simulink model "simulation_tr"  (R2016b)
settings: Solver=ode45  StartTime=0.0  StopTime=35*3600  RelTol=1e-3  EnableMultiTasking=on
undefined symbols (not defined in the file or in its folder): C0, C1, drhe, drhi, dte, dti, dto, Icc, Nbre, Qair, Qpanne, R_iso, serial, V, V0, V1
libraries: powerlib_meascontrol x4, instrumentlib x3, simulink x1

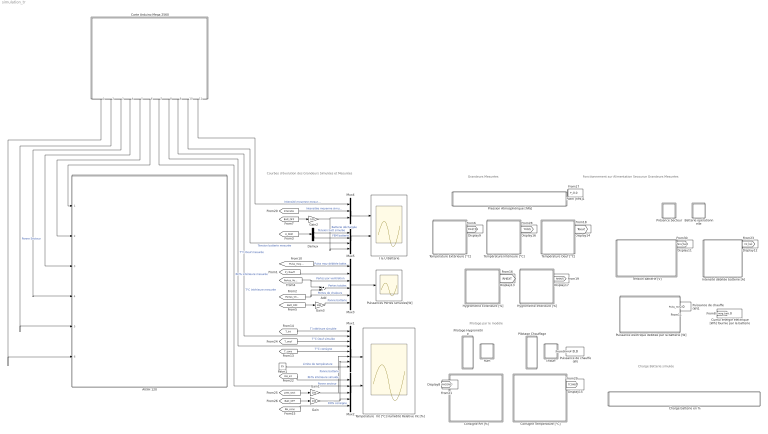
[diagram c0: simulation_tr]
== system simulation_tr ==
  note: Fonctionnement sur Alimentation Secourue Grandeurs Mesurées
  note: Grandeurs Mesurées
  note: Pilotage par le modèle
  note: Courbes d'évolution des Grandeurs Simulées et Mesurées
  note: Charge Batterie simulée
  AVXH 120 : Subsystem
  Add : Sum
  Batterie opérationnelle : Subsystem  DialogController=hmiCreateDDGDialog  IsWebBlock=on
  Carte Arduino Mega 2560 : Subsystem
  Charge batterie en % : Subsystem  DialogController=hmiCreateDDGDialog  IsWebBlock=on
  Consigne RH [%] : Subsystem  DialogController=hmiCreateDDGDialog  IsWebBlock=on
  Consigne Température [°C] : Subsystem  DialogController=hmiCreateDDGDialog  IsWebBlock=on
  Cumul énergie électrique [Wh] fournie par la batterie : Display
  Demux : Demux  Outputs=2
  Display{8..9,11..17} (9 alike) : Display
  Gain{,1..3} (4 alike) : Gain  Gain=100
  Hygrométrie Extérieure [%] : Subsystem  DialogController=hmiCreateDDGDialog  IsWebBlock=on
  Hygrométrie Intérieure [%] : Subsystem  DialogController=hmiCreateDDGDialog  IsWebBlock=on
  I & U Batterie : Scope  NumInputPorts=2
  Intensité débitée batterie [A] : Subsystem  DialogController=hmiCreateDDGDialog  IsWebBlock=on
  Mux1 : Mux  Inputs=8
  Mux2 : Mux  Inputs=5
  Mux3 : Mux  Inputs=6
  Mux4 : Mux  Inputs=3
  Mux5 : Mux
  Patm [hPa]1 : Display
  Patm1 : Constant  Value=25
  Pilotage Chauffage : Subsystem  DialogController=hmiCreateDDGDialog  IsWebBlock=on
  Pilotage Hygrométrie : Subsystem  DialogController=hmiCreateDDGDialog  IsWebBlock=on
  Pression Atmosphérique [hPa] : Subsystem  DialogController=hmiCreateDDGDialog  IsWebBlock=on
  Présence Secteur : Subsystem  DialogController=hmiCreateDDGDialog  IsWebBlock=on
  Puissance de chauffe (W) : Display
  Puissance de chauffe (W)1 : Display
  Puissance électrique débitée par la batterie [W] : Subsystem  DialogController=hmiCreateDDGDialog  IsWebBlock=on
  Puissances Pertes simulées[W] : Scope
  Température Extérieure [°C] : Subsystem  DialogController=hmiCreateDDGDialog  IsWebBlock=on
  Température Intérieure [°C] : Subsystem  DialogController=hmiCreateDDGDialog  IsWebBlock=on
  Température  Int [°C] Humidité Relative Int [%] : Scope  NumInputPorts=2
  Température Oeuf [°C] : Subsystem  DialogController=hmiCreateDDGDialog  IsWebBlock=on
  Tension batterie [V] : Subsystem  DialogController=hmiCreateDDGDialog  IsWebBlock=on
  chauff : Subsystem  DialogController=hmiCreateDDGDialog  IsWebBlock=on
  hum : Subsystem  DialogController=hmiCreateDDGDialog  IsWebBlock=on
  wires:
  [T_int] -> Mux1/1  "T intérieure simulée"
  [Intensite] -> Mux4/2  "Intensitée moyenne simulée"
  [RH_int] -> Mux2/1  "RH% intérieure simulée"
  Gain1/1 -> Mux1/6, Mux2/3  "Panne secteur"
  [pres_sect] -> Gain1/1
  [Batt_OFF] -> Gain/1
  Gain/1 -> Mux1/7, Mux2/4  "Panne batterie"
  Demux/1 -> Mux5/1  "Tension batt simulée"
  [T_cons] -> Mux1/5  "T°C consigne"
  Carte Arduino Mega 2560/1(Patm) -> AVXH 120/6(In6)
  Mux1/1 -> Température  Int [°C] Humidité Relative Int [%]/1
  Mux2/1 -> Température  Int [°C] Humidité Relative Int [%]/2
  [P_chauff] -> Mux3/2
  [Pertes_Vent] -> Mux3/3, Add/1  "Pertes par ventilation"
  Mux3/1 -> Puissances Pertes simulées[W]/1
  [Pertes_Chaleur] -> Mux3/5, Add/2  "Pertes de chaleurs"
  Add/1 -> Mux3/4  "Pertes totales"
  [T_oeuf] -> Mux1/3  "T°C Oeuf simulée"
  Carte Arduino Mega 2560/9(T°C INT) -> Mux1/2  "T°C intérieure mesurée"
  Carte Arduino Mega 2560/7(RH% INT) -> Mux2/2  "RH% intérieure mesurée"
  Carte Arduino Mega 2560/4(RH% EXT) -> AVXH 120/3(In4)
  Carte Arduino Mega 2560/3(T°C EXT) -> AVXH 120/4(In5)
  Carte Arduino Mega 2560/2(Pres Sect) -> AVXH 120/5(Présence secteur)  "Panne Secteur"
  [RH_cons] -> Mux2/5  "RH% consigne"
  Carte Arduino Mega 2560/8(T°C OEUF) -> Mux1/4  "T°C Oeuf mesurée"
  Carte Arduino Mega 2560/5(RH Cons) -> AVXH 120/2(In3)
  Carte Arduino Mega 2560/6(T°C Cons) -> AVXH 120/1(In2)
  [RHCONS] -> Display8/1
  [TCONS] -> Display15/1
  [TCINT] -> Display16/1
  [P_atm] -> Patm [hPa]1/1
  [TCEXT] -> Display9/1
  [Toeuf] -> Display14/1
  [RHINT] -> Display17/1
  [RHEXT] -> Display13/1
  [Int_bat] -> Display12/1
  [Tens_bat] -> Display11/1
  Mux4/1 -> I & U Batterie/1
  Mux5/1 -> I & U Batterie/2
  Carte Arduino Mega 2560/10(U) -> Mux5/3  "Tension batterie mesurée"
  [U_FEM] -> Demux/1
  Demux/2 -> Mux5/2  "FEM batterie"
  [Batt_OFF] -> Gain2/1
  Gain2/1 -> Mux5/4, Mux4/3  "Batterie déchargée"
  [Batt_OFF] -> Gain3/1
  Gain3/1 -> Mux3/6  "Panne batterie"
  [Energ_batt] -> Cumul énergie électrique [Wh] fournie par la batterie/1
  Carte Arduino Mega 2560/11(Imoy) -> Mux4/1  "Intensité moyenne mesurée"
  [Puiss_moy_debitee] -> Mux3/1  "Puiss moy débitée batterie mesurée"
  Patm1/1 -> Mux1/8  "Limite de température"
  [PCHAUFF] -> Puissance de chauffe (W)/1
  [Puiss_moy_debitee] -> Puissance de chauffe (W)1/1

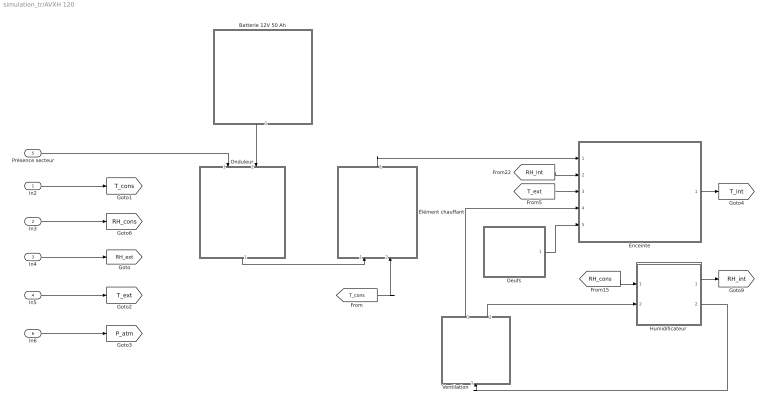
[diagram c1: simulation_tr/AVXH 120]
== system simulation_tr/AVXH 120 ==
  In2 : Inport
  In3 : Inport  Port=2
  In4 : Inport  Port=3
  In5 : Inport  Port=4
  Présence secteur : Inport  Port=5
  In6 : Inport  Port=6
  Batterie 12V 50 Ah : Subsystem
  Enceinte : Subsystem
  Humidificateur : Subsystem
  Oeufs : Subsystem
  Onduleur : Subsystem
  Ventilation : Subsystem
  Élément chauffant : Subsystem
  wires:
  [RH_int] -> Enceinte/2(In2)
  Enceinte/1(T°C in) -> [T_int]
  Présence secteur/1 -> Onduleur/1(In1)
  In6/1 -> [P_atm]
  In5/1 -> [T_ext]
  [T_ext] -> Enceinte/3(T°C ext)
  In4/1 -> [RH_ext]
  In3/1 -> [RH_cons]
  Oeufs/1(Out1) -> Enceinte/5(M.Cp_Oeuf)
  Élément chauffant/1(Out2) -> Enceinte/1(P_chauff)
  Ventilation/1(Out1) -> Enceinte/4(Pertes ventilation)
  [RH_cons] -> Humidificateur/1(In1)
  Ventilation/2(Out2) -> Humidificateur/2(In2)
  Humidificateur/2(Out2) -> Ventilation/1(In1)
  In2/1 -> [T_cons]
  Batterie 12V 50 Ah/1(Out3) -> Onduleur/2(In2)
  Onduleur/1(Out1) -> Élément chauffant/1(In1)
  [T_cons] -> Élément chauffant/2(In2)
  Humidificateur/1(Out1) -> [RH_int]

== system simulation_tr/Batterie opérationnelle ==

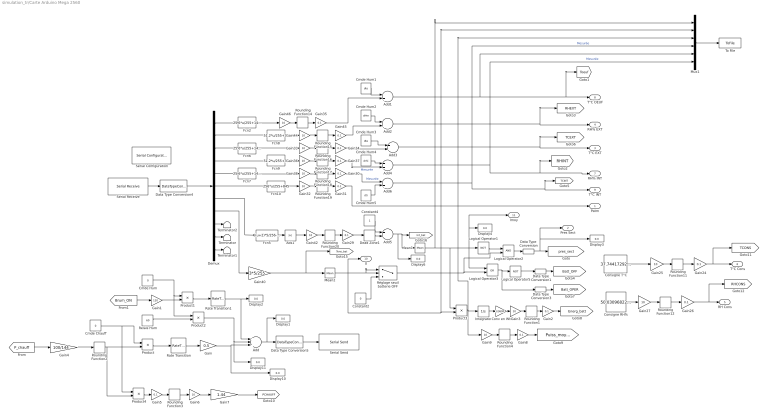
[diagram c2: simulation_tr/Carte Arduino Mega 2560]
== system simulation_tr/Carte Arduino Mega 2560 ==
  Abs1 : Abs
  Add : Sum  Inputs=+++
  Add{1..6} (6 alike) : Sum
  Cmde Chauff : Constant  Value=0  SampleTime=1
  Cmde Hum : Constant  Value=0  SampleTime=1
  Cmde Hum1 : Constant  Value=dto  SampleTime=1
  Cmde Hum2 : Constant  Value=drhe  SampleTime=1
  Cmde Hum3 : Constant  Value=dte  SampleTime=1
  Cmde Hum4 : Constant  Value=drhi  SampleTime=1
  Cmde Hum5 : Constant  Value=dti  SampleTime=1
  Consigne RH% : Constant  Value=50.030968221029
  Consigne T°C : Constant  Value=37.74417292277
  Constant2 : Constant  Value=0
  Constant4 : Constant
  Conv en Wh : Gain  Gain=1/3600
  Data Type Conversion{,1,3..4} (4 alike) : DataTypeConversion  OutDataTypeStr=double
  Data Type Conversion5 : DataTypeConversion  OutDataTypeStr=uint8
  Dead Zone1 : DeadZone  LowerValue=0  UpperValue=1
  Demux : Demux  Outputs=11
  Display{1..4,6,10..11} (7 alike) : Display
  Fcn10 : Fcn  Expr=256*u/255+845
  Fcn2 : Fcn  Expr=25.6*u/255+14.4
  Fcn5 : Fcn  Expr=((u+2)*5/256-2.5)/0.0833
  Fcn6 : Fcn  Expr=25.6*u/255+14.4
  Fcn7 : Fcn  Expr=25.6*u/255+14.4
  Fcn8 : Fcn  Expr=51.2*u/255+35
  Fcn9 : Fcn  Expr=51.2*u/255+35
  Gain : Gain  Gain=0.5
  Gain1 : Gain  Gain=120
  Gain{2,5,8,24,26,29..31,34..35,37,45} (12 alike) : Gain  Gain=0.1
  Gain{3,6,9,25,27,32..33,36,38,42,44,46} (12 alike) : Gain  Gain=10
  Gain4 : Gain  Gain=100/144
  Gain40 : Gain  Gain=3*5/255
  Gain7 : Gain  Gain=1.44
  Integrator : Integrator
  Logical Operator1 : Logic  Operator=NOT  AllPortsSameDT=off  OutDataTypeStr=boolean
  Logical Operator2 : Logic  AllPortsSameDT=off  OutDataTypeStr=boolean
  Logical Operator3 : Logic  Operator=OR  AllPortsSameDT=off  OutDataTypeStr=boolean
  Logical Operator5 : Logic  Operator=NOT  AllPortsSameDT=off  OutDataTypeStr=boolean
  Mean1 : powerlib_meascontrol/Measurements/Mean  Freq=0.1  Vinit=0  Ts=1
  Mean2 : powerlib_meascontrol/Measurements/Mean  Freq=0.1  Vinit=0  Ts=1
  Mux1 : Mux  Inputs=6
  Product{,1..4} (5 alike) : Product
  Rate Transition : RateTransition  OutPortSampleTime=1
  Rate Transition1 : RateTransition  OutPortSampleTime=1
  Relais Hum : Constant  Value=60  SampleTime=1
  Rounding Function{1..4,11..12,14..20} (13 alike) : Rounding  Operator=round
  Réglage seuil batterie OFF : Switch  Criteria=u2 > Threshold  Threshold=11.5
  Serial Configuration : instrumentlib/Serial Configuration  Priority=-200000  ComPortMenu=<Please select a port...>  ComPort=COM8  ObjConstructor=serial('COM8');  BaudRate=9600  DataBits=8  Parity=none  StopBits=1  FlowControl=none  Timeout=10  ByteOrder=LittleEndian
  Serial Receive : instrumentlib/Serial Receive  ComPortMenu=<Please select a port...>  ComPort=COM8  ObjConstructor=serial('COM8');  Terminator=<none>  DataSize="[1  11]"  DataType=uint8  EnableBlockingMode=on  ActionDataUnavailable=Output last received value  CustomValue=0  SampleTime=1
  Serial Send : instrumentlib/Serial Send  ComPortMenu=<Please select a port...>  ComPort=COM8  ObjConstructor=serial('COM8');  Terminator=<none>  EnableBlockingMode=on
  Terminator : Terminator
  Terminator1 : Terminator
  Terminator2 : Terminator
  To File : ToFile  Filename=mesures.mat  SaveFormat=Timeseries
  Patm : Outport
  Pres Sect : Outport  Port=2
  T°C EXT : Outport  Port=3
  RH% EXT : Outport  Port=4
  RH Cons : Outport  Port=5
  T°C Cons : Outport  Port=6
  RH% INT : Outport  Port=7
  T°C OEUF : Outport  Port=8
  T°C INT : Outport  Port=9
  U : Outport  Port=10
  Imoy : Outport  Port=11
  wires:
  Rounding Function11/1 -> Gain24/1
  Gain25/1 -> Rounding Function11/1
  Consigne T°C/1 -> Gain25/1
  Gain24/1 -> [TCONS], T°C Cons/1
  Rounding Function12/1 -> Gain26/1
  Gain27/1 -> Rounding Function12/1
  Gain26/1 -> [RHCONS], RH Cons/1
  Consigne RH%/1 -> Gain27/1
  Mux1/1 -> To File/1
  Add1/1 -> Mux1/5, [Toeuf], T°C OEUF/1
  Add2/1 -> [RHEXT], RH% EXT/1
  Gain31/1 -> Patm/1
  Demux/7 -> Fcn5/1
  Add4/1 -> Mux1/6, RH% INT/1, [RHINT]  "Mesurée"
  Add3/1 -> T°C EXT/1, [TCEXT]
  Gain40/1 -> Mean2/1, [Tens_bat]
  Demux/2 -> Fcn8/1
  Demux/3 -> Fcn6/1
  Demux/4 -> Fcn9/1
  Demux/5 -> Fcn7/1
  Demux/1 -> Fcn2/1
  Fcn2/1 -> Gain46/1
  Fcn6/1 -> Gain33/1
  Fcn7/1 -> Gain38/1
  Fcn8/1 -> Gain44/1
  Fcn9/1 -> Gain36/1
  Fcn10/1 -> Gain32/1
  Rounding Function14/1 -> Gain35/1
  Gain46/1 -> Rounding Function14/1
  Rounding Function15/1 -> Gain45/1
  Gain44/1 -> Rounding Function15/1
  Rounding Function16/1 -> Gain34/1
  Gain33/1 -> Rounding Function16/1
  Rounding Function17/1 -> Gain37/1
  Gain36/1 -> Rounding Function17/1
  Rounding Function18/1 -> Gain30/1
  Gain38/1 -> Rounding Function18/1
  Rounding Function19/1 -> Gain31/1
  Gain32/1 -> Rounding Function19/1
  Serial Receive/1 -> Data Type Conversion4/1
  Data Type Conversion4/1 -> Demux/1
  Rounding Function20/1 -> Gain29/1
  Gain42/1 -> Rounding Function20/1
  Demux/6 -> Fcn10/1
  Add6/1 -> Mux1/4, T°C INT/1, [TCINT]  "Mesurée"
  Fcn5/1 -> Abs1/1
  Gain/1 -> Display10/1, Add/3
  Demux/10 -> Terminator/1
  Demux/11 -> Terminator1/1
  Demux/9 -> Terminator2/1
  Data Type Conversion5/1 -> Serial Send/1
  Rate Transition/1 -> Gain/1
  Constant2/1 -> Réglage seuil batterie OFF/3
  Demux/8 -> Gain40/1
  Réglage seuil batterie OFF/1 -> Logical Operator3/2, Logical Operator2/2
  Data Type Conversion/1 -> Pres Sect/1, Display3/1, [pres_sect]
  Add5/1 -> Display6/1, Mean1/1, [Int_bat]
  Cmde Chauff/1 -> Product4/1, Product/1
  Product/1 -> Rate Transition/1
  Logical Operator2/1 -> Data Type Conversion/1
  Logical Operator3/1 -> Data Type Conversion3/1, Logical Operator5/1
  Logical Operator5/1 -> Data Type Conversion1/1
  Logical Operator1/1 -> Logical Operator2/1
  Data Type Conversion1/1 -> [Batt_OFF]
  Data Type Conversion3/1 -> [Batt_OPER]
  [P_chauff] -> Gain4/1
  Add/1 -> Display1/1, Data Type Conversion5/1
  Cmde Hum/1 -> Product2/1, Product1/1
  [Brum_ON] -> Gain1/1
  Gain1/1 -> Product1/2
  Product1/1 -> Rate Transition1/1
  Rate Transition1/1 -> Display2/1, Add/1
  Relais Hum/1 -> Product2/2
  Product2/1 -> Display11/1, Add/2
  Product3/1 -> Mux1/3, Gain9/1, Integrator/1
  Integrator/1 -> Conv en Wh/1
  Conv en Wh/1 -> Gain3/1
  Rounding Function1/1 -> Gain2/1
  Gain3/1 -> Rounding Function1/1
  Gain2/1 -> [Energ_batt]
  Abs1/1 -> Gain42/1
  Mean1/1 -> Imoy/1, Display4/1, Logical Operator3/1, Logical Operator1/1, Product3/1, Mux1/1
  Mean2/1 -> Réglage seuil batterie OFF/2, Réglage seuil batterie OFF/1, Mux1/2, Product3/2, U/1
  Gain4/1 -> Rounding Function2/1
  Rounding Function2/1 -> Product4/2, Product/2
  Gain5/1 -> Rounding Function3/1
  Rounding Function3/1 -> Gain6/1
  Gain6/1 -> Gain7/1
  Cmde Hum1/1 -> Add1/1
  Gain35/1 -> Add1/2
  Cmde Hum2/1 -> Add2/1
  Gain45/1 -> Add2/2
  Cmde Hum3/1 -> Add3/1
  Gain34/1 -> Add3/2
  Cmde Hum4/1 -> Add4/1
  Gain37/1 -> Add4/2  "Mesurée"
  Cmde Hum5/1 -> Add6/2
  Gain30/1 -> Add6/1  "Mesurée"
  Gain7/1 -> [PCHAUFF]
  Product4/1 -> Gain5/1
  Dead Zone1/1 -> Add5/2
  Constant4/1 -> Add5/1
  Rounding Function4/1 -> Gain8/1
  Gain9/1 -> Rounding Function4/1
  Gain8/1 -> [Puiss_moy_debitee]
  Gain29/1 -> Dead Zone1/1

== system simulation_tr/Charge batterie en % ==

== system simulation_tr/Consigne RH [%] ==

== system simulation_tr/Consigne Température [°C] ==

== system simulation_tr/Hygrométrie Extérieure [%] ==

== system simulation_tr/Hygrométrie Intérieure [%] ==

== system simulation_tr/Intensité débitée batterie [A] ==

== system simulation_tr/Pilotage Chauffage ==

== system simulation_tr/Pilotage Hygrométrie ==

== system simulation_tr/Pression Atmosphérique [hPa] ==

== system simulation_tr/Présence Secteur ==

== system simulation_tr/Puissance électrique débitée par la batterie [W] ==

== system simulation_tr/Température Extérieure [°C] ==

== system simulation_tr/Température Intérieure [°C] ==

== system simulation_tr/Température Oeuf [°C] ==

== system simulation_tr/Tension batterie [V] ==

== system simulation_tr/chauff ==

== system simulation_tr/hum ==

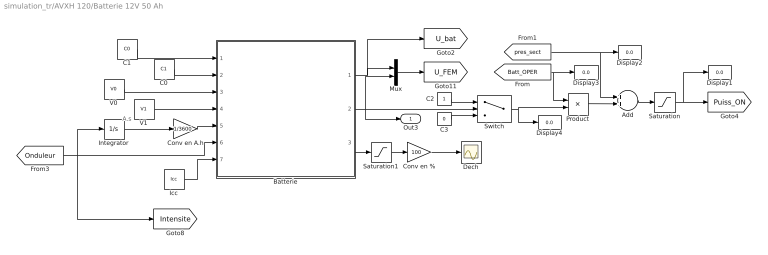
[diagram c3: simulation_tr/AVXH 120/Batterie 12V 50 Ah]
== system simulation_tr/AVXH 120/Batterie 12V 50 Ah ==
  note: A.s
  Add : Sum
  Batterie : MATLAB Function  TreatAsAtomicUnit=on
  C0 : Constant  Value=C1
  C1 : Constant  Value=C0
  C2 : Constant
  C3 : Constant  Value=0
  Conv en % : Gain  Gain=100
  Conv en A.h : Gain  Gain=1/3600
  Dech : Scope
  Display{1..4} (4 alike) : Display
  Icc : Constant  Value=Icc
  Integrator : Integrator
  Mux : Mux  Inputs=2
  Product : Product
  Saturation : Saturate  UpperLimit=1  LowerLimit=0
  Saturation1 : Saturate  UpperLimit=1000  LowerLimit=0
  Switch : Switch  Criteria=u2 > Threshold  Threshold=11
  V0 : Constant  Value=V0
  V1 : Constant  Value=V1
  Out3 : Outport
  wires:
  Batterie/3(x) -> Saturation1/1
  Conv en %/1 -> Dech/1
  Batterie/1(U) -> [U_bat], Mux/1
  C0/1 -> Batterie/2(C1)
  C1/1 -> Batterie/1(C0)
  V0/1 -> Batterie/3(V0)
  V1/1 -> Batterie/4(V1)
  Icc/1 -> Batterie/7(Icc)
  Integrator/1 -> Conv en A.h/1
  Conv en A.h/1 -> Batterie/5(C)
  Mux/1 -> [U_FEM]
  C2/1 -> Switch/1
  C3/1 -> Switch/3
  Saturation1/1 -> Conv en %/1
  Switch/1 -> Display4/1, Product/2
  Product/1 -> Add/2
  [Batt_OPER] -> Display3/1, Product/1
  Add/1 -> Saturation/1
  [pres_sect] -> Display2/1, Add/1
  Batterie/2(E) -> Mux/2, Out3/1, Switch/2
  Saturation/1 -> Display1/1, [Puiss_ON]
  [Onduleur] -> [Intensite], Integrator/1, Batterie/6(I)

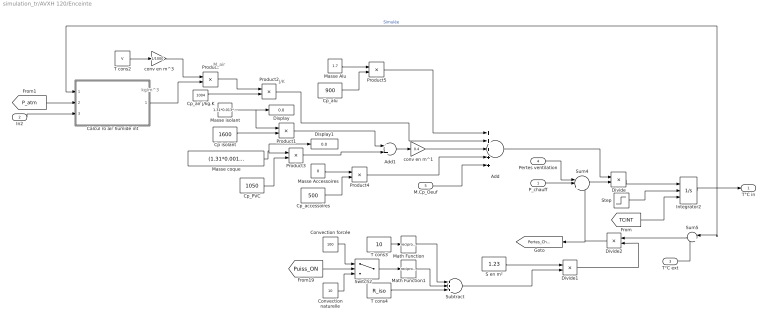
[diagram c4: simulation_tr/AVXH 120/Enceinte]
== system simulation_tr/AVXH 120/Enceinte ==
  note: J/K
  note: kg/m^3
  note: M_air
  P_chauff : Inport
  In2 : Inport  Port=2
  T°C ext : Inport  Port=3
  Pertes ventilation : Inport  Port=4
  M.Cp_Oeuf : Inport  Port=5
  Add : Sum  Inputs=+++++
  Add1 : Sum
  Calcul ro air humide int : MATLAB Function  TreatAsAtomicUnit=on
  Convection forcée : Constant  Value=100
  Convection naturelle : Constant  Value=10
  Cp isolant : Constant  Value=1600
  Cp_PVC : Constant  Value=1050
  Cp_accessoires : Constant  Value=500
  Cp_air j/kg.K : Constant  Value=1004
  Cp_alu : Constant  Value=900
  Display : Display
  Display1 : Display
  Divide : Product  Inputs=/*
  Divide1 : Product  Inputs=*/
  Divide2 : Product  Inputs=**
  Integrator2 : Integrator  ExternalReset=rising  InitialConditionSource=external  InitialCondition=20
  Masse Accessoires : Constant  Value=8
  Masse Alu : Constant  Value=1.7
  Masse coque : Constant  Value=(1.31*0.001+1.23*0.001)*1380
  Masse isolant : Constant  Value=1.31*0.013*40
  Math Function : Math  Operator=reciprocal
  Math Function1 : Math  Operator=reciprocal
  Product{,1..5} (6 alike) : Product
  S en m² : Constant  Value=1.23
  Step : Step  SampleTime=0
  Subtract : Sum  Inputs=+++
  Sum4 : Sum  Inputs=-|+|-
  Sum5 : Sum  Inputs=|+-
  Switch2 : Switch  Criteria=u2 > Threshold
  T cons2 : Constant  Value=V
  T cons3 : Constant  Value=10
  T cons4 : Constant  Value=R_iso
  conv en m^1 : Gain  Gain=0.4
  conv en m^3 : Gain  Gain=1/1000
  T°C in : Outport
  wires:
  P_chauff/1 -> Sum4/2
  Sum4/1 -> Divide/2
  Sum5/1 -> Divide2/1
  Divide2/1 -> Sum4/3, [Pertes_Chaleur]
  Divide/1 -> Integrator2/1
  T°C ext/1 -> Sum5/2
  T cons2/1 -> conv en m^3/1
  Calcul ro air humide int/1(RO) -> Product/2
  Product/1 -> Product2/1
  Masse isolant/1 -> Display/1, Product1/1
  Cp_air j/kg.K/1 -> Product2/2
  Cp isolant/1 -> Product1/2
  Product1/1 -> Add1/1
  Product2/1 -> Add/2
  [P_atm] -> Calcul ro air humide int/2(P)
  Add/1 -> Divide/1
  S en m²/1 -> Divide1/1
  T cons4/1 -> Subtract/3
  Divide1/1 -> Divide2/2
  In2/1 -> Calcul ro air humide int/3(RH)
  Pertes ventilation/1 -> Sum4/1
  conv en m^3/1 -> Product/1
  T cons3/1 -> Math Function/1
  Switch2/1 -> Math Function1/1
  Math Function1/1 -> Subtract/2
  Math Function/1 -> Subtract/1
  Subtract/1 -> Divide1/2
  Cp_PVC/1 -> Product3/2
  Product3/1 -> Add1/2
  Masse Accessoires/1 -> Product4/1
  Cp_accessoires/1 -> Product4/2
  Product4/1 -> Add/4
  Masse Alu/1 -> Product5/1
  Cp_alu/1 -> Product5/2
  Product5/1 -> Add/1
  M.Cp_Oeuf/1 -> Add/5
  [TCINT] -> Integrator2/3
  Masse coque/1 -> Display1/1, Product3/1
  Integrator2/1 -> Sum5/1, Calcul ro air humide int/1(T), T°C in/1  "Simulée"
  Add1/1 -> conv en m^1/1
  conv en m^1/1 -> Add/3
  Convection forcée/1 -> Switch2/1
  Convection naturelle/1 -> Switch2/3
  [Puiss_ON] -> Switch2/2
  Step/1 -> Integrator2/2

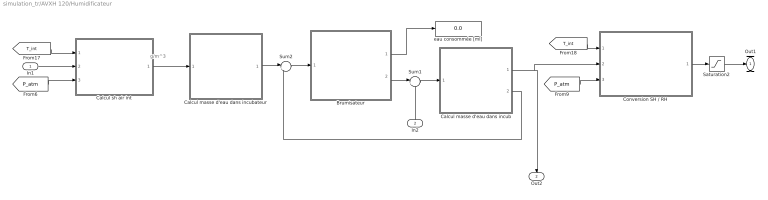
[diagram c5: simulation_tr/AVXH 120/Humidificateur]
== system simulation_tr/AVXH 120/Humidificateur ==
  note: g/m^3
  In1 : Inport
  In2 : Inport  Port=2
  Brumisateur : Subsystem
  Calcul masse d'eau dans incub : Subsystem
  Calcul masse d'eau dans incubateur : Subsystem
  Calcul sh air int : MATLAB Function  TreatAsAtomicUnit=on
  Conversion SH / RH : MATLAB Function  TreatAsAtomicUnit=on
  Saturation2 : Saturate  UpperLimit=100  LowerLimit=0
  Sum1 : Sum  Inputs=|++
  Sum2 : Sum  Inputs=|+-
  eau consommée [ml] : Display
  Out1 : Outport
  Out2 : Outport  Port=2
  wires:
  Sum2/1 -> Brumisateur/1(In1)
  [P_atm] -> Calcul sh air int/3(pl)
  Conversion SH / RH/1(rh) -> Saturation2/1
  Brumisateur/2(Out2) -> Sum1/1
  In1/1 -> Calcul sh air int/2(rh)
  Calcul sh air int/1(sh) -> Calcul masse d'eau dans incubateur/1(In1)
  Calcul masse d'eau dans incub/1(Out1) -> Out2/1, Conversion SH / RH/2(sh)
  Sum1/1 -> Calcul masse d'eau dans incub/1(In1)
  [T_int] -> Calcul sh air int/1(T)
  Calcul masse d'eau dans incubateur/1(Out1) -> Sum2/1
  In2/1 -> Sum1/2
  [T_int] -> Conversion SH / RH/1(T)
  [P_atm] -> Conversion SH / RH/3(pl)
  Brumisateur/1(Q eau consommée (ml)) -> eau consommée [ml]/1
  Calcul masse d'eau dans incub/2(Out2) -> Sum2/2
  Saturation2/1 -> Out1/1

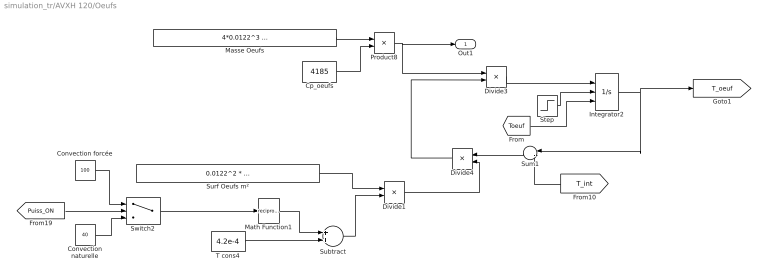
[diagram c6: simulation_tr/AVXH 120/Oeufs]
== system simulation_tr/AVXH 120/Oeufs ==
  Convection forcée : Constant  Value=100
  Convection naturelle : Constant  Value=40
  Cp_oeufs : Constant  Value=4185
  Divide1 : Product  Inputs=*/
  Divide3 : Product  Inputs=/*
  Divide4 : Product  Inputs=**
  Integrator2 : Integrator  ExternalReset=rising  InitialConditionSource=external  InitialCondition=20
  Masse Oeufs : Constant  Value=4*0.0122^3 * (3.14 * (3 - 1.4142) - 1) * 1000 * Nbre / 3
  Math Function1 : Math  Operator=reciprocal
  Product8 : Product
  Step : Step  SampleTime=0
  Subtract : Sum
  Sum1 : Sum  Inputs=|-+
  Surf Oeufs m² : Constant  Value=0.0122^2 * (3.14 * (3 - 1.4142) - 1) * Nbre
  Switch2 : Switch  Criteria=u2 > Threshold  Threshold=0.5
  T cons4 : Constant  Value=4.2e-4
  Out1 : Outport
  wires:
  Cp_oeufs/1 -> Product8/2
  Masse Oeufs/1 -> Product8/1
  Product8/1 -> Out1/1, Divide3/1
  Divide4/1 -> Divide3/2
  [Toeuf] -> Integrator2/3
  Integrator2/1 -> [T_oeuf], Sum1/1
  Sum1/1 -> Divide4/1
  T cons4/1 -> Subtract/2
  Divide1/1 -> Divide4/2
  Math Function1/1 -> Subtract/1
  Subtract/1 -> Divide1/2
  [T_int] -> Sum1/2
  Divide3/1 -> Integrator2/1
  Surf Oeufs m²/1 -> Divide1/1
  Convection forcée/1 -> Switch2/1
  Convection naturelle/1 -> Switch2/3
  [Puiss_ON] -> Switch2/2
  Switch2/1 -> Math Function1/1
  Step/1 -> Integrator2/2

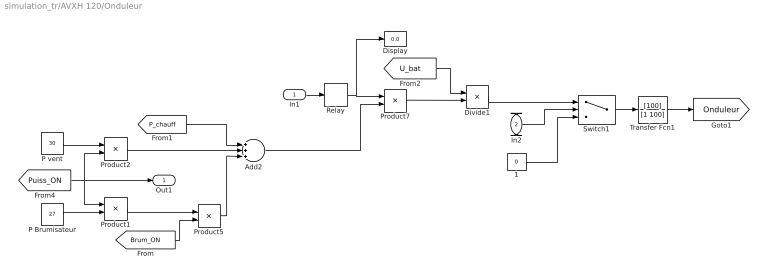
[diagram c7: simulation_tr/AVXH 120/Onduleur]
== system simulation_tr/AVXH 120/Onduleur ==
  In1 : Inport
  In2 : Inport  Port=2
  1 : Constant  Value=0
  Add2 : Sum  Inputs=+++
  Display : Display
  Divide1 : Product  Inputs=/*
  P Brumisateur : Constant  Value=27
  P vent : Constant  Value=30
  Product{1..2,5,7} (4 alike) : Product
  Relay : Relay  OnSwitchValue=1  OffSwitchValue=0  OnOutputValue=0  OffOutputValue=1
  Switch1 : Switch  Threshold=11
  Transfer Fcn1 : TransferFcn  Numerator=[100]  Denominator=[1 100]
  Out1 : Outport
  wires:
  Relay/1 -> Display/1, Product7/1
  Add2/1 -> Product7/2
  Product2/1 -> Add2/2
  [Brum_ON] -> Product5/2
  P Brumisateur/1 -> Product1/2
  Product5/1 -> Add2/3
  In1/1 -> Relay/1
  [P_chauff] -> Add2/1
  Divide1/1 -> Switch1/1
  1/1 -> Switch1/3
  Product7/1 -> Divide1/2
  [U_bat] -> Divide1/1
  Switch1/1 -> Transfer Fcn1/1
  In2/1 -> Switch1/2
  [Puiss_ON] -> Product1/1, Out1/1, Product2/2
  Product1/1 -> Product5/1
  P vent/1 -> Product2/1
  Transfer Fcn1/1 -> [Onduleur]

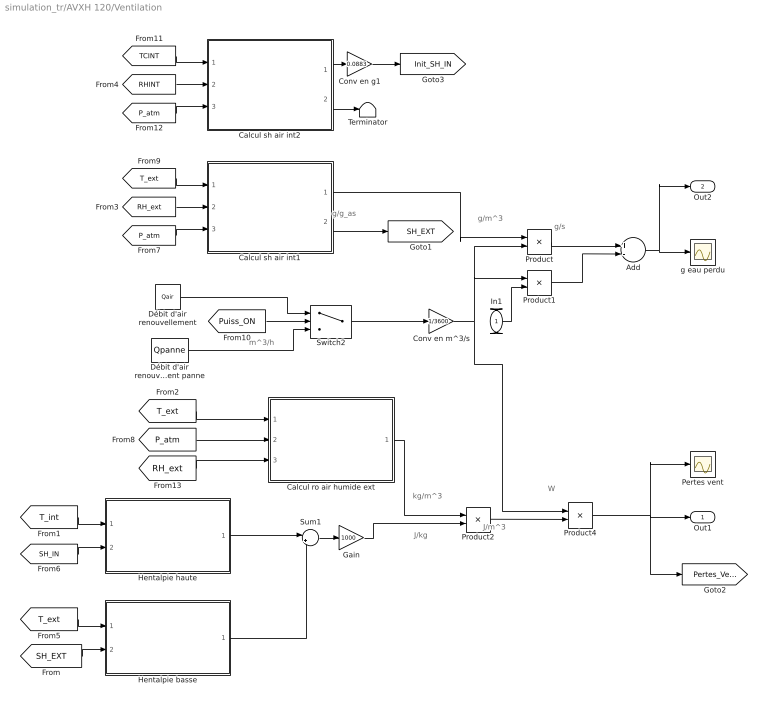
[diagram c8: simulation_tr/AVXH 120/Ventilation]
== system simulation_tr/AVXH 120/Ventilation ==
  note: g/g_as
  note: g/s
  note: W
  note: J/m^3
  note: kg/m^3
  note: J/kg
  note: g/m^3
  note: m^3/h
  In1 : Inport
  Add : Sum  Inputs=+-
  Calcul ro air humide ext : MATLAB Function  TreatAsAtomicUnit=on
  Calcul sh air int1 : MATLAB Function  TreatAsAtomicUnit=on
  Calcul sh air int2 : MATLAB Function  TreatAsAtomicUnit=on
  Conv en g1 : Gain  Gain=0.0883
  Conv en m^3/s : Gain  Gain=1/3600
  Débit d'air renouvellement : Constant  Value=Qair
  Débit d'air renouvellement panne : Constant  Value=Qpanne
  Gain : Gain  Gain=1000
  Hentalpie basse : MATLAB Function  TreatAsAtomicUnit=on
  Hentalpie haute : MATLAB Function  TreatAsAtomicUnit=on
  Pertes vent : Scope
  Product{,1..2,4} (4 alike) : Product
  Sum1 : Sum  Inputs=|+-
  Switch2 : Switch  Criteria=u2 > Threshold
  Terminator : Terminator
  g eau perdu : Scope
  Out1 : Outport
  Out2 : Outport  Port=2
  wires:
  Add/1 -> Out2/1, g eau perdu/1
  Switch2/1 -> Conv en m^3/s/1
  Conv en m^3/s/1 -> Product1/1, Product/2, Product4/1
  Product/1 -> Add/1
  Product1/1 -> Add/2
  Calcul ro air humide ext/1(RO) -> Product2/1
  Product2/1 -> Product4/2
  Débit d'air renouvellement/1 -> Switch2/1
  Débit d'air renouvellement panne/1 -> Switch2/3
  [Puiss_ON] -> Switch2/2
  [T_ext] -> Calcul ro air humide ext/1(T)
  [T_ext] -> Calcul sh air int1/1(T)
  [P_atm] -> Calcul sh air int1/3(pl)
  [P_atm] -> Calcul ro air humide ext/2(P)
  [RH_ext] -> Calcul sh air int1/2(rh)
  [RH_ext] -> Calcul ro air humide ext/3(RH)
  Product4/1 -> [Pertes_Vent], Out1/1, Pertes vent/1
  In1/1 -> Product1/2
  Gain/1 -> Product2/2
  [T_int] -> Hentalpie haute/1(T)
  [T_ext] -> Hentalpie basse/1(T)
  [SH_EXT] -> Hentalpie basse/2(SH)
  [SH_IN] -> Hentalpie haute/2(SH)
  Hentalpie haute/1(H1) -> Sum1/1
  Hentalpie basse/1(H1) -> Sum1/2
  Sum1/1 -> Gain/1
  Calcul sh air int1/2(sh2) -> [SH_EXT]
  [RHINT] -> Calcul sh air int2/2(rh)
  [TCINT] -> Calcul sh air int2/1(T)
  [P_atm] -> Calcul sh air int2/3(pl)
  Calcul sh air int2/1(sh) -> Conv en g1/1
  Conv en g1/1 -> [Init_SH_IN]
  Calcul sh air int1/1(sh) -> Product/1
  Calcul sh air int2/2(sh2) -> Terminator/1

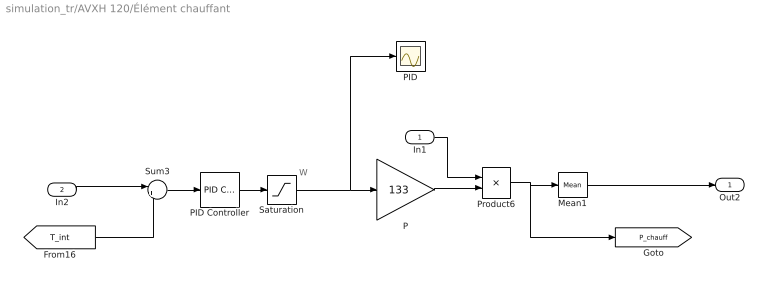
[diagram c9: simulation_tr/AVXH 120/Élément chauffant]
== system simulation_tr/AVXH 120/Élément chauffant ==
  note: W
  In1 : Inport
  In2 : Inport  Port=2
  Mean1 : powerlib_meascontrol/Measurements/Mean  Freq=0.1  Vinit=0  Ts=1
  P : Gain  Gain=133
  PID : Scope
  PID Controller : simulink/Continuous/PID Controller  Controller=PID  TimeDomain=Continuous-time  SampleTime=-1  IntegratorMethod=Forward Euler  FilterMethod=Forward Euler  Form=Parallel  UseFilter=on  ControllerParametersSource=internal  P=0.0897573355031779  I=3.41688472569394e-05  D=-22.2891464593491  N=0.00402695256486726  InitialConditionSource=internal  InitialConditionForIntegrator=0  InitialConditionForFilter=0  ExternalReset=none  LimitOutput=off  UpperSaturationLimit=inf  LowerSaturationLimit=-inf  LinearizeAsGain=on  AntiWindupMode=none  Kb=1  TrackingMode=off  Kt=1  PParamMin=[]  PParamMax=[]  IParamMin=[]  IParamMax=[]  DParamMin=[]  DParamMax=[]  NParamMin=[]  NParamMax=[]  KbParamMin=[]  KbParamMax=[]  KtParamMin=[]  KtParamMax=[]  POutMin=[]  POutMax=[]  IOutMin=[]  IOutMax=[]  DOutMin=[]  DOutMax=[]  NOutMin=[]  NOutMax=[]  KbOutMin=[]  KbOutMax=[]  KtOutMin=[]  KtOutMax=[]  IntegratorOutMin=[]  IntegratorOutMax=[]  FilterOutMin=[]  FilterOutMax=[]  SumOutMin=[]  SumOutMax=[]  SumI1OutMin=[]  SumI1OutMax=[]  SumI2OutMin=[]  SumI2OutMax=[]  SumI3OutMin=[]  SumI3OutMax=[]  SumDOutMin=[]  SumDOutMax=[]  SaturationOutMin=[]  SaturationOutMax=[]  IntegratorContinuousStateAttributes=''  IntegratorStateMustResolveToSignalObject=off  IntegratorRTWStateStorageClass=Auto  FilterContinuousStateAttributes=''  FilterStateMustResolveToSignalObject=off  FilterRTWStateStorageClass=Auto  DifferentiatorICPrevScaledInput=0  DifferentiatorOutMin=[]  DifferentiatorOutMax=[]
  Product6 : Product
  Saturation : Saturate  UpperLimit=1  LowerLimit=0
  Sum3 : Sum  Inputs=|+-
  Out2 : Outport
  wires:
  In2/1 -> Sum3/1
  PID Controller/1 -> Saturation/1
  Sum3/1 -> PID Controller/1
  Product6/1 -> Mean1/1, [P_chauff]
  [T_int] -> Sum3/2
  In1/1 -> Product6/1
  P/1 -> Product6/2
  Saturation/1 -> P/1, PID/1
  Mean1/1 -> Out2/1

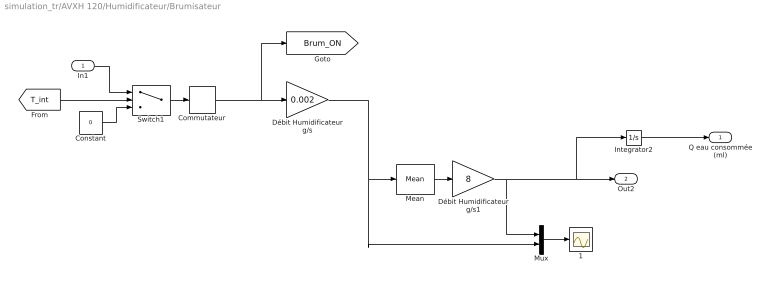
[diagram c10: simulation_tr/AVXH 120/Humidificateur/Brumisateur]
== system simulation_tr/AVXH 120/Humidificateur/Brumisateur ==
  In1 : Inport
  1 : Scope
  Commutateur : Relay  OnSwitchValue=0.11  OffSwitchValue=-0.02
  Constant : Constant  Value=0
  Débit Humidificateur g/s : Gain  Gain=0.002
  Débit Humidificateur g/s1 : Gain  Gain=8
  Integrator2 : Integrator
  Mean : powerlib_meascontrol/Measurements/Mean  Freq=0.061  Vinit=0  Ts=0
  Mux : Mux  Inputs=2
  Switch1 : Switch  Criteria=u2 > Threshold  Threshold=25
  Q eau consommée (ml) : Outport
  Out2 : Outport  Port=2
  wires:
  Integrator2/1 -> Q eau consommée (ml)/1
  Commutateur/1 -> Débit Humidificateur g/s/1, [Brum_ON]
  In1/1 -> Switch1/1
  Débit Humidificateur g/s/1 -> Mux/2, Mean/1
  Mux/1 -> 1/1
  Mean/1 -> Débit Humidificateur g/s1/1
  Débit Humidificateur g/s1/1 -> Mux/1, Integrator2/1, Out2/1
  Switch1/1 -> Commutateur/1
  [T_int] -> Switch1/2
  Constant/1 -> Switch1/3

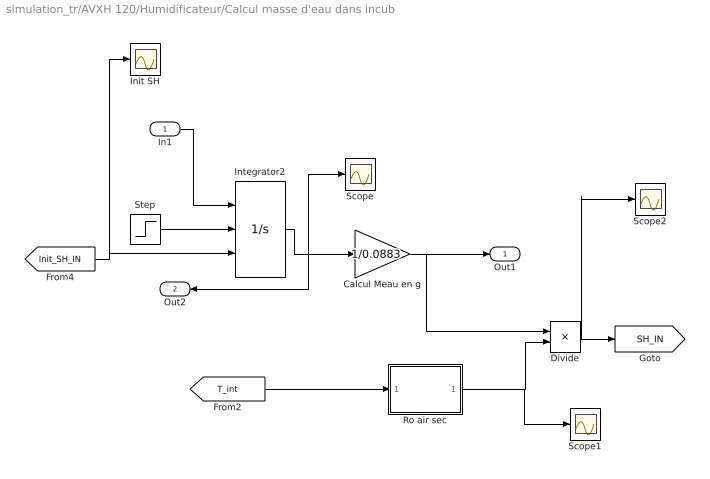
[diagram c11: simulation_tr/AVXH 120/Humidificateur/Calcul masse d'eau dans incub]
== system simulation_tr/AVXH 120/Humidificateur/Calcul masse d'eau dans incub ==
  In1 : Inport
  Calcul Meau en g : Gain  Gain=1/0.0883
  Divide : Product  Inputs=*/
  Init SH : Scope
  Integrator2 : Integrator  ExternalReset=rising  InitialConditionSource=external  InitialCondition=1
  Ro air sec : MATLAB Function  TreatAsAtomicUnit=on
  Scope : Scope
  Scope1 : Scope
  Scope2 : Scope
  Step : Step  SampleTime=0
  Out1 : Outport
  Out2 : Outport  Port=2
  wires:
  Calcul Meau en g/1 -> Divide/1, Out1/1
  In1/1 -> Integrator2/1
  Integrator2/1 -> Scope/1, Calcul Meau en g/1, Out2/1
  Ro air sec/1(ro) -> Scope1/1, Divide/2
  [T_int] -> Ro air sec/1(T)
  Divide/1 -> Scope2/1, [SH_IN]
  [Init_SH_IN] -> Init SH/1, Integrator2/3
  Step/1 -> Integrator2/2

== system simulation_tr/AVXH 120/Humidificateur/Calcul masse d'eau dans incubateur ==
  In1 : Inport
  Calcul Masse eau dans Incub en g : Gain  Gain=0.0883
  Out1 : Outport
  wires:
  In1/1 -> Calcul Masse eau dans Incub en g/1
  Calcul Masse eau dans Incub en g/1 -> Out1/1

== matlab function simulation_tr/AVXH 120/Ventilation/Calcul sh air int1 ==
function [sh,sh2] =CONV_RH_en_SH(T,rh,pl)

% ######################################################################################################
% function [sh]=goff_gratch(T,rh,pl)
%
% fonction de conversion de l'humidité relative ('rh' : en %)
% en humidité spécifique ('sh' : en g/m^3)
% en fonction de :
% la temperature de l'air ('T' : Kelvin, utiliser la fonction C2K si la T est en °C)
% du niveau pression ('pl' : en hPa, si vous avez des matrices 4D, bouclez sur la dimension 
% niveau). 
%
% utilise l'equation de Goff-Gratch pour la determination de
% la tension de vapeur saturante (es) en fonction de la temperature de l'Air
%
% AUTHOR : Nicolas Fauchereau - CRC Dijon - <nicolasf@u-bourgogne.fr>
%
% ######################################################################################################



%Conversion température
T=T+273;


% tension de vapeur saturante
if (T<0), % par rapport a la glace 
eilog = -9.09718 .* ((273.16 ./ T) -1);
eilog2 = -3.5654 .* log10 (273.16 ./ T);
eilog3 = 0.876793 .* (1 - (T ./ 273.16 ));
es=6.1071 .* 10.^(eilog+eilog2+eilog3);

else, % par rapport à l'eau 
eilog=-7.90298 .* ((373.16 ./ T) - 1);
eilog2=5.02808 .* log10((373.16 ./ T));
eilog3=-1.3816e-7 .* ((10.^(11.344.*(1-(T./373.16)))) -1);
eilog4=8.1328e-3 .* ((10.^( -3.49149 .* ((373.16 ./ T) - 1) )) -1);
es=1013.246 .* 10.^(eilog+eilog2+eilog3+eilog4);
end;


% masse
ws = 0.62197 .* es ./ (pl - 0.378.*es);

% masse volumique
ro = 1.293 .* 273 ./ (T);

% humidité spécifique
sh2 = (rh/100.0) .* ws*1000;
sh=sh2*ro; %%% passage en g.m^3

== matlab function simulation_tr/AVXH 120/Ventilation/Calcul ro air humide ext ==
function RO = RO_AIR_HUMIDE(T,P,RH)
P=P*100;
RH=RH/100;
RO = 1/(287.06*(T+273.15))*(P-230.617*RH*exp(17.5043*T/(241.2+T)));

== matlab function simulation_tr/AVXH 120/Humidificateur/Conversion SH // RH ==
function rh  = CONV_SH_en_RH(T,sh,pl)

% ######################################################################################################
% function [sh]=goff_gratch_shtorh(T,sh,pl)
%
% fonction de conversion de l'humidité spécifique ('sh' : en g/m^3)
% en humidité relative ('rh' : %)
% en fonction de :
% la temperature de l'air ('T' : Kelvin, utiliser la fonction C2K si la T est en °C)
% du niveau pression ('pl' : en hPa, si vous avez des matrices 4D, bouclez sur la dimension
% niveau).
%
% utilise l'equation de Goff-Gratch pour la determination de
% la tension de vapeur saturante (es) en fonction de la temperature de l'Air
%
% AUTHOR : Nicolas Fauchereau - CRC Dijon - <nicolasf@u-bourgogne.fr>
%
% ######################################################################################################

%Conversion température
T=T+273;

% tension de vapeur saturante
%if (K2C(T)<0), % par rapport a la glace
if (T<0),
eilog = -9.09718 .* ((273.16 ./ T) -1);
eilog2 = -3.5654 .* log10 (273.16 ./ T);
eilog3 = 0.876793 .* (1 - (T ./ 273.16 ));
es=6.1071 .* 10.^(eilog+eilog2+eilog3);

else, % par rapport à l'eau
eilog=-7.90298 .* ((373.16 ./ T) - 1);
eilog2=5.02808 .* log10((373.16 ./ T));
eilog3=-1.3816e-7 .* ((10.^(11.344.*(1-(T./373.16)))) -1);
eilog4=8.1328e-3 .* ((10.^( -3.49149 .* ((373.16 ./ T) - 1) )) -1);
es=1013.246 .* 10.^(eilog+eilog2+eilog3+eilog4);
end;


% masse
ws = 0.62197 .* es ./ (pl - 0.378.*es);

% masse volumique
ro = 1.293 .* 273 ./ (T);

% humidité relative
rh=(sh./ws) .* 100/(1000*ro);

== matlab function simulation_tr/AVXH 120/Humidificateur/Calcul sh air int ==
function sh =CONV_RH_en_SH(T,rh,pl)

% ######################################################################################################
% function [sh]=goff_gratch(T,rh,pl)
%
% fonction de conversion de l'humidité relative ('rh' : en %)
% en humidité spécifique ('sh' : en g/m^3)
% en fonction de :
% la temperature de l'air ('T' : Kelvin, utiliser la fonction C2K si la T est en °C)
% du niveau pression ('pl' : en hPa, si vous avez des matrices 4D, bouclez sur la dimension 
% niveau). 
%
% utilise l'equation de Goff-Gratch pour la determination de
% la tension de vapeur saturante (es) en fonction de la temperature de l'Air
%
% AUTHOR : Nicolas Fauchereau - CRC Dijon - <nicolasf@u-bourgogne.fr>
%
% ######################################################################################################



%Conversion température
T=T+273.2;


% tension de vapeur saturante
if (T<0), % par rapport a la glace 
eilog = -9.09718 .* ((273.16 ./ T) -1);
eilog2 = -3.5654 .* log10 (273.16 ./ T);
eilog3 = 0.876793 .* (1 - (T ./ 273.16 ));
es=6.1071 .* 10.^(eilog+eilog2+eilog3);

else, % par rapport à l'eau 
eilog=-7.90298 .* ((373.16 ./ T) - 1);
eilog2=5.02808 .* log10((373.16 ./ T));
eilog3=-1.3816e-7 .* ((10.^(11.344.*(1-(T./373.16)))) -1);
eilog4=8.1328e-3 .* ((10.^( -3.49149 .* ((373.16 ./ T) - 1) )) -1);
es=1013.246 .* 10.^(eilog+eilog2+eilog3+eilog4);
end;


% masse
ws = 0.62197 .* es ./ (pl - 0.378.*es);

% masse volumique
ro = 1.293 .* 273 ./ (T);

% humidité spécifique
sh = (rh/100.0)*ws;
sh=sh*1000*ro; %%% passage en g.m^3

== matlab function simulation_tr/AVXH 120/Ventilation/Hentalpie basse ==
function H1 = CALC_HENTALP(T,SH)

H1 =1.006*T+SH*(2500+1.826*T)/1000;

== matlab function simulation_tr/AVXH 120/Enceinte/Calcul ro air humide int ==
function RO = F(T,P,RH)
P=P*100;
RH=RH/100;
RO = 1/(287.06*(T+273.15))*(P-230.617*RH*exp(17.5043*T/(241.2+T)));

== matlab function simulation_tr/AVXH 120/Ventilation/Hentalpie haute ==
function H1 = CALC_HENTALP(T,SH)

H1 =1.006*T+SH*(2500+1.826*T)/1000;

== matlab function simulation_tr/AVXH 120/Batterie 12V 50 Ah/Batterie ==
function [U,E,x] = Batterie(C0, C1, V0, V1, C,I, Icc)
%#codegen


x1=C1/C0;
B=(V1-x1*V0)/(V1*(1-x1));
A=1-B;
x=(C0-C)/C0;
V = V0*(1-(A*(1-x))/(1-B*(1-x)));
U=V-V*I/Icc;
E = U/(1-I/Icc);

== matlab function simulation_tr/AVXH 120/Humidificateur/Calcul masse
d'eau dans incub/Ro air sec ==
function ro = fcn(T)
%#codegen
T=T+273.15;
ro = 1.293 .* 273 ./ (T);

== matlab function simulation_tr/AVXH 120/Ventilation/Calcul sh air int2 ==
function [sh,sh2] =CONV_RH_en_SH(T,rh,pl)

% ######################################################################################################
% function [sh]=goff_gratch(T,rh,pl)
%
% fonction de conversion de l'humidité relative ('rh' : en %)
% en humidité spécifique ('sh' : en g/m^3)
% en fonction de :
% la temperature de l'air ('T' : Kelvin, utiliser la fonction C2K si la T est en °C)
% du niveau pression ('pl' : en hPa, si vous avez des matrices 4D, bouclez sur la dimension 
% niveau). 
%
% utilise l'equation de Goff-Gratch pour la determination de
% la tension de vapeur saturante (es) en fonction de la temperature de l'Air
%
% AUTHOR : Nicolas Fauchereau - CRC Dijon - <nicolasf@u-bourgogne.fr>
%
% ######################################################################################################



%Conversion température
T=T+273;


% tension de vapeur saturante
if (T<0), % par rapport a la glace 
eilog = -9.09718 .* ((273.16 ./ T) -1);
eilog2 = -3.5654 .* log10 (273.16 ./ T);
eilog3 = 0.876793 .* (1 - (T ./ 273.16 ));
es=6.1071 .* 10.^(eilog+eilog2+eilog3);

else, % par rapport à l'eau 
eilog=-7.90298 .* ((373.16 ./ T) - 1);
eilog2=5.02808 .* log10((373.16 ./ T));
eilog3=-1.3816e-7 .* ((10.^(11.344.*(1-(T./373.16)))) -1);
eilog4=8.1328e-3 .* ((10.^( -3.49149 .* ((373.16 ./ T) - 1) )) -1);
es=1013.246 .* 10.^(eilog+eilog2+eilog3+eilog4);
end;


% masse
ws = 0.62197 .* es ./ (pl - 0.378.*es);

% masse volumique
ro = 1.293 .* 273 ./ (T);

% humidité spécifique
sh2 = (rh/100.0) .* ws*1000;
sh=sh2*ro; %%% passage en g.m^3
